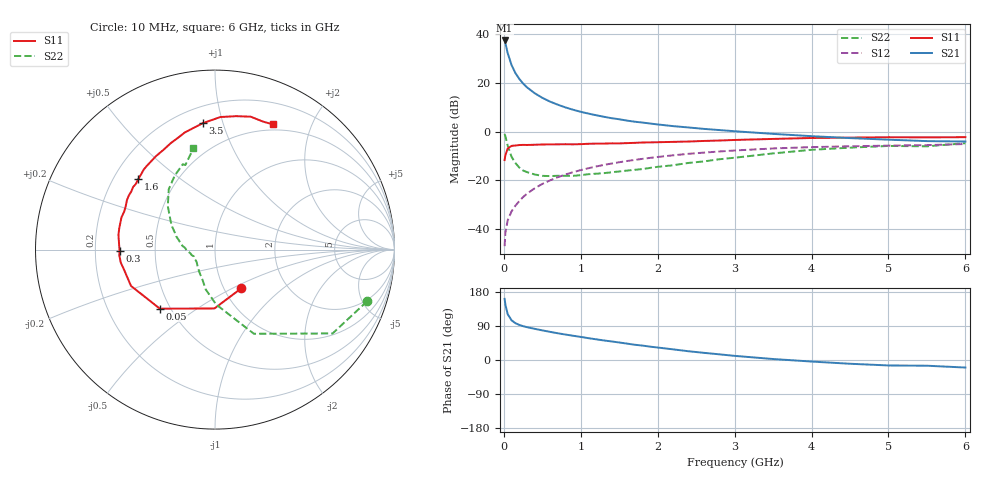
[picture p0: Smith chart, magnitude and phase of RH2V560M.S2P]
! SIEMENS Small Signal Semiconductors
! BFR106
! Si NPN RF Bipolar Junction Transistor in SOT23
! VCE = 2.5 V  IC = 60 mA
! Common Emitter S-Parameters:  August  1996
# GHz  S  MA  R  50
!  f  S11  S21  S12  S22
! GHz  MAG  ANG  MAG  ANG  MAG  ANG  MAG  ANG
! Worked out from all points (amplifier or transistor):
!   36 points, 10 MHz to 6 GHz, reference 50 ohm
!   highest |S21| = 37.3 dB at 10 MHz (marker M1)
!   |S21| within 3 dB of that: start of sweep to 34.07 MHz
!   unconditionally stable (mu >= 1): 219.4 MHz to 2.629 GHz; 5.288 GHz to end of sweep
!   at 250 MHz: K = 1.02, MAG = 22.3 dB, |S12| = -26.8 dB
!   at 1.4 GHz: K = 1.06, MAG = 7.8 dB, |S12| = -13.1 dB
!   at 6 GHz: K = 1.00, MAG = 0.3 dB, |S12| = -5.1 dB
!   S11 on the Smith chart (normalised r, x): 10 MHz: 1.20, -0.56; 50 MHz: 0.44, -0.36; 300 MHz: 0.31, -0.00; 1.6 GHz: 0.30, +0.36; 3.5 GHz: 0.31, +0.86; 6 GHz: 0.43, +1.47
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0.01  0.2608 -55.7  73.53 161.3  0.0045 77.3  0.8949 -18.8
0.02  0.3279 -90.5  64.82 146.5  0.0085 66.8  0.8045 -35.5
0.05  0.4502 -133.0  40.6 120.9  0.0152 60.6  0.5166 -65.2
0.1  0.5098 -156.6  23.09 104.8  0.0232 62.7  0.3058 -88.8
0.15  0.5186 -167.3  15.83 97.2  0.0303 65.7  0.2273 -103.3
0.2  0.5301 -172.2  12.06 92.7  0.0376 68.6  0.1842 -111.9
0.25  0.5341 -176.6  9.652 89.3  0.0456 70.0  0.1595 -121.3
0.3  0.5319 -179.4  8.084 86.7  0.0534 71.8  0.1482 -127.2
0.4  0.5373 175.2  6.118 82.3  0.0689 71.9  0.1324 -137.7
0.5  0.5441 171.3  4.917 78.2  0.0846 71.8  0.124 -145.2
0.6  0.5466 167.5  4.115 74.3  0.1002 71.2  0.1227 -149.7
0.7  0.5482 164.0  3.562 70.6  0.1162 70.2  0.1244 -154.2
0.8  0.5512 161.0  3.13 67.2  0.1321 68.7  0.1244 -159.0
1.1  0.5628 150.7  2.336 57.6  0.1777 64.6  0.134 -166.9
1.3  0.5678 145.3  2.012 51.6  0.2076 61.3  0.1408 -172.6
1.6  0.5806 137.4  1.679 43.3  0.2497 56.5  0.1589 -179.3
2.2  0.6157 122.4  1.294 28.1  0.3266 46.5  0.2045 166.4
2.8  0.6557 108.4  1.075 15.0  0.391 36.7  0.2711 151.8
3.5  0.7073 95.6  0.898 2.6  0.4513 25.8  0.3572 137.4
4.5  0.7527 81.0  0.736 -9.9  0.4997 11.5  0.4691 118.6
5.5  0.7618 69.4  0.638 -15.1  0.528 2.6  0.4993 109.3
6  0.7681 65.3  0.626 -19.9  0.5565 -4.2  0.5773 102.0
